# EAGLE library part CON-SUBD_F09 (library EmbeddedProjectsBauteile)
SUB-D 9pins
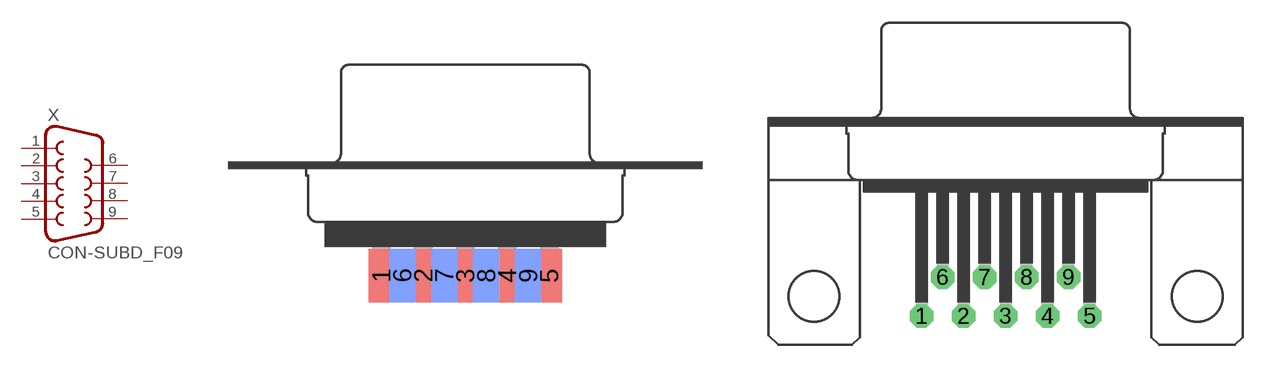
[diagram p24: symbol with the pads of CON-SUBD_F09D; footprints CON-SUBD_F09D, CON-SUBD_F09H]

Designator prefix X

## CON-SUBD_F09D (EP: 400506)  [CON-SUBD_F09D]
1  1  pas
2  2  pas
3  3  pas
4  4  pas
5  5  pas
6  6  pas
7  7  pas
8  8  pas
9  9  pas

## CON-SUBD_F09H  [CON-SUBD_F09H]
Pads as for CON-SUBD_F09D

## CON-SUBD_F09HP  [CON-SUBD_F09HP]
Pads as for CON-SUBD_F09D

## Footprint CON-SUBD_F09D (pad centres in mm)
smd 1.7 x 3.5: 1 -5.486,-6.045; 2 -2.743,-6.045; 3 0,-6.045; 4 2.743,-6.045; 5 5.486,-6.045
smd 1.7 x 3.5 bottom: 6 -4.115,-6.045; 7 -1.372,-6.045; 8 1.372,-6.045; 9 4.115,-6.045

## Footprint CON-SUBD_F09H (pad centres in mm)
drill 1.016 octagon: 1 -5.486,-1.27; 2 -2.743,-1.27; 3 0,-1.27; 4 2.743,-1.27; 5 5.486,-1.27; 6 -4.115,1.27; 7 -1.372,1.27; 8 1.372,1.27; 9 4.115,1.27
hole 3.302 at -12.522,0
hole 3.302 at 12.522,0

## Footprint CON-SUBD_F09HP (pad centres in mm)
drill 1.016 octagon: 1 -5.486,-1.27; 2 -2.743,-1.27; 3 0,-1.27; 4 2.743,-1.27; 5 5.486,-1.27; 6 -4.115,1.27; 7 -1.372,1.27; 8 1.372,1.27; 9 4.115,1.27
drill 3.302 pad 5.08: G1 -12.522,0; G2 12.522,0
